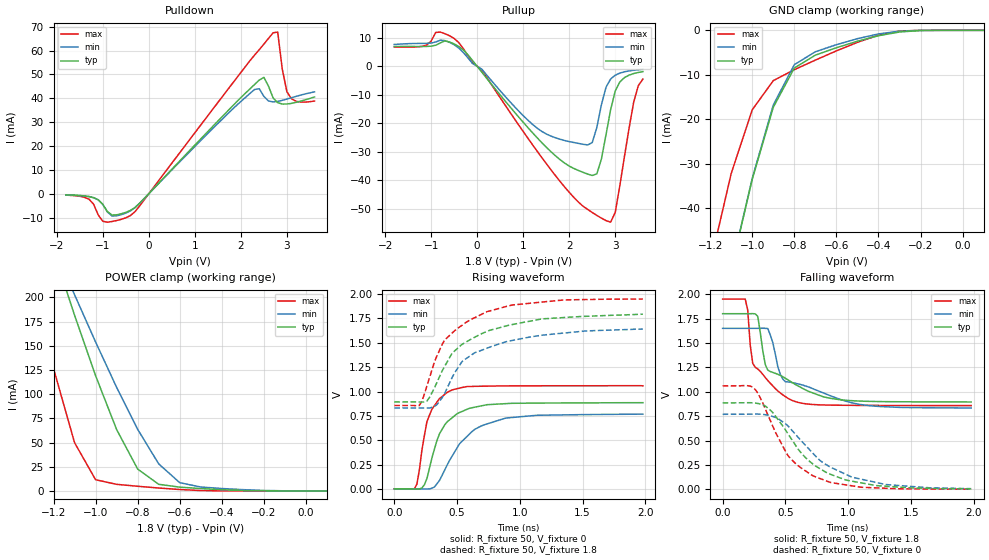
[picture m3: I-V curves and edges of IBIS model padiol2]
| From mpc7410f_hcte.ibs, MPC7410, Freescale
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| *   padiol2 Model   *
[Model]   padiol2
Model_type   I/O
Polarity   Non-Inverting
Vinl = 0.63V
Vinh = 1.17V
Vmeas = 0.9V
Cref = 0
Rref = 50
Vref = 0.9V
|   typ   min   max
C_comp   3.887100e-12   3.331920e-12   4.126430e-12
|   typ   min   max
[Voltage range]   1.8V   1.65V   1.95V
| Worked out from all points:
|   slope of the pulldown table from 0 to 0.27 V, typ, clamps not added: 48.8 ohm
|   slope of the pullup table from 0 to 0.27 V, typ, clamps not added: 49.4 ohm
|   GND clamp passes 1 mA (typ) near -0.37 V on its own axis
|   POWER clamp passes 1 mA (typ) near -0.37 V on its own axis
|   falling waveform, R_fixture 50, V_fixture 1.8: 20-80 % time 278ps typ, 382ps min, 182ps max; typ from 1.8 V to 0.896 V
|   rising waveform, R_fixture 50, V_fixture 0: 20-80 % time 167ps typ, 259ps min, 114ps max; typ from 0.005 V to 0.887 V
|   falling waveform, R_fixture 50, V_fixture 0: 20-80 % time 371ps typ, 428ps min, 300ps max; typ from 0.887 V to 0.005 V
|   rising waveform, R_fixture 50, V_fixture 1.8: 20-80 % time 399ps typ, 408ps min, 334ps max; typ from 0.894 V to 1.79 V
[Pulldown]
|   Voltage   I(typ)   I(min)   I(max)
-1.8V     -485.4uA   -500.5uA   -592.6uA
-1.3V     -1.192mA   -1.218mA   -2.295mA
-1V       -4.458mA   -4.481mA   -11.55mA
-800mV    -8.932mA   -9.322mA   -11.65mA
-400mV    -6.998mA   -7.209mA   -9.163mA
2.4V      47.66mA    44.01mA    60.4mA
2.5V      48.78mA    40.81mA    62.73mA
2.7V      40.17mA    38.49mA    67.45mA
2.8V      38.17mA    38.69mA    67.75mA
2.9V      37.59mA    39.14mA    52.15mA
3V        37.59mA    39.67mA    42.74mA
3.6V      40.54mA    42.69mA    38.84mA
[GND_clamp]
-1.8V     -241mA     -241mA     -217.6mA
-1.2V     -76.28mA   -76.24mA   -52.5mA
-1.1V     -53.65mA   -53.55mA   -32.15mA
-1V       -33.47mA   -33.24mA   -17.84mA
-900mV    -17.29mA   -16.78mA   -11.3mA
-800mV    -8.472mA   -7.715mA   -8.846mA
-700mV    -5.574mA   -4.816mA   -6.69mA
-500mV    -2.448mA   -1.876mA   -2.696mA
-400mV    -1.215mA   -809.5uA   -1.086mA
-300mV    -374.2uA   -188.3uA   -155.1uA
-200mV    -45.6uA    -17.29uA   -4.047uA
100mV     0A         0A         0A
[Pullup]
-1.8V     6.905mA    7.648mA    6.733mA
-1.1V     6.949mA    8.046mA    7.427mA
-900mV    7.38mA     8.513mA    11.86mA
-500mV    7.853mA    7.56mA     9.75mA
1.4V      -26.67mA   -22.77mA   -31.87mA
2.5V      -38.25mA   -26.73mA   -51.2mA
2.6V      -37.67mA   -21.43mA   -52.23mA
2.7V      -32.44mA   -13.45mA   -53.19mA
2.9V      -15.17mA   -4.449mA   -54.61mA
3V        -8.627mA   -3.112mA   -51.16mA
3.4V      -2.538mA   -1.391mA   -12.65mA
3.6V      -1.863mA   -1.049mA   -4.496mA
[POWER_clamp]
-1.8V     669.5mA    563.8mA    715.3mA
-1.3V     315.6mA    303.6mA    216.7mA
-1.2V     247.5mA    252.7mA    126.5mA
-1.1V     181.5mA    202.7mA    49.83mA
-1V       119mA      153.9mA    11.58mA
-900mV    63.41mA    107mA      6.793mA
-800mV    22.61mA    63.64mA    4.804mA
-700mV    6.839mA    27.96mA    3.007mA
-600mV    3.906mA    8.511mA    1.457mA
-500mV    2.44mA     4.04mA     390.9uA
-400mV    1.258mA    2.498mA    33.33uA
100mV     0A         0A         0A
|   typ   min   max
[Ramp]
dV/dt_r   0.52922/1.66542e-10   0.45866/2.59168e-10   0.63464/1.14402e-10
dV/dt_f   0.54339/2.79660e-10   0.49050/3.83022e-10   0.65524/1.81524e-10
[Falling Waveform]
R_fixture = 50
V_fixture = 1.8
V_fixture_min = 1.65
V_fixture_max = 1.95
| time   V(typ)   V(min)   V(max)
0s        1.8V       1.65V      1.95V
180ps     1.8V       1.65V      1.95V
200ps     1.8V       1.65V      1.836V
240ps     1.801V     1.65V      1.291V
280ps     1.772V     1.65V      1.233V
360ps     1.222V     1.648V     1.115V
460ps     1.168V     1.178V     987.3mV
560ps     1.09V      1.092V     908.4mV
1.12ns    903.6mV    865.6mV    860.4mV
1.98ns    895.6mV    834.2mV    858.5mV
[Rising Waveform]
R_fixture = 50
V_fixture = 0
V_fixture_min = 0
V_fixture_max = 0
| time   V(typ)   V(min)   V(max)
0s        4.676mV    4.857mV    3.26mV
160ps     2.955mV    3.77mV     5.012mV
180ps     2.519mV    3.666mV    52.02mV
220ps     13.11mV    2.663mV    399.7mV
260ps     109.4mV    2.552mV    691.8mV
360ps     567.4mV    89.58mV    927.6mV
460ps     731.2mV    337.6mV    1.016V
640ps     840.4mV    612.3mV    1.054V
880ps     876.2mV    726.1mV    1.058V
1.98ns    886.6mV    769.1mV    1.059V
[Falling Waveform]
R_fixture = 50
V_fixture = 0
V_fixture_min = 0
V_fixture_max = 0
| time   V(typ)   V(min)   V(max)
0s        886.7mV    769.3mV    1.059V
260ps     884.2mV    771.8mV    1.022V
380ps     812.1mV    755.7mV    705.4mV
520ps     570.9mV    651.7mV    347.2mV
620ps     382.6mV    506.6mV    224.3mV
720ps     258.8mV    369mV      138.2mV
840ps     163.8mV    241.6mV    80.31mV
1.04ns    81.68mV    122.6mV    34.32mV
1.3ns     32.17mV    49.48mV    11.28mV
1.98ns    4.786mV    7.225mV    2.156mV
[Rising Waveform]
R_fixture = 50
V_fixture = 1.8
V_fixture_min = 1.65
V_fixture_max = 1.95
| time   V(typ)   V(min)   V(max)
0s        894.3mV    832.5mV    857.9mV
200ps     893.4mV    832.3mV    857.9mV
280ps     939.2mV    831.2mV    1.14V
340ps     1.095V     866.9mV    1.367V
400ps     1.256V     977.9mV    1.527V
460ps     1.392V     1.143V     1.599V
540ps     1.484V     1.308V     1.68V
740ps     1.618V     1.446V     1.82V
1.18ns    1.745V     1.578V     1.918V
1.98ns    1.793V     1.641V     1.948V
